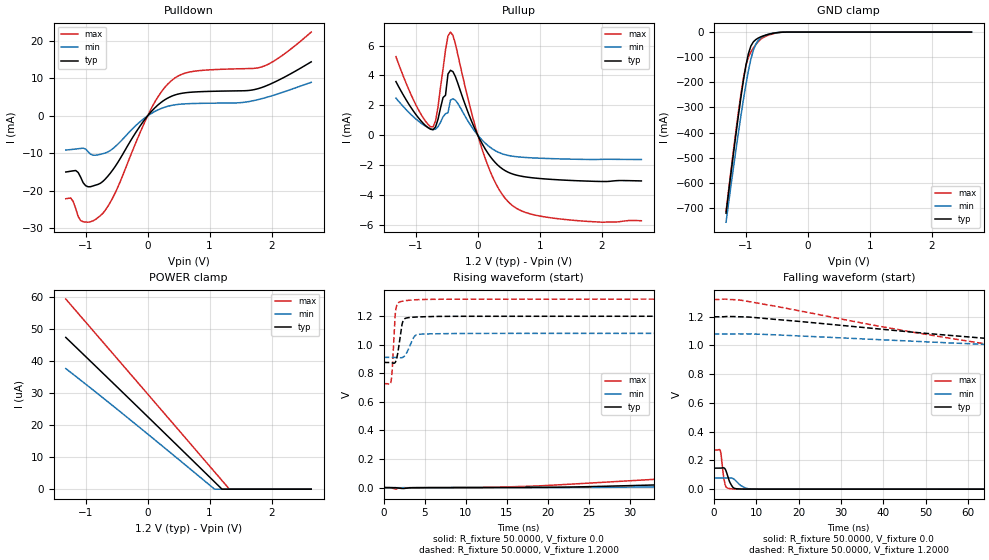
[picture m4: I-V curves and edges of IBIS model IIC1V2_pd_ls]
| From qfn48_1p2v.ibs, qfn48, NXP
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[Model] IIC1V2_pd_ls
|   Model IIC1V2_pd_ls
| This model was characterised for following simulation conditions:
| External (pad) voltage:
|   - Typ: 1.2V,   - Min: 1.08V,   - Max: 1.32V
| Library cells for typ/min/max conditions are connected as defined below:
|  IO - External Pad
|  A - Core Input
|  EN - Output Buffer Enable
|  BOOST - vdde
|  EGP - vdd
|  EHS - gnd
|  ENZI - vdd
|  EPD - vdd
|  EPUN - vdd
|  ZI - NC
|  ZIF - NC
|  gnd - gnd
|  gnde - gnde
|  vdd - vdd
|  vdde - vdde
| All other pins connected to ground
Model_type I/O
Polarity   Non-Inverting
Enable   Active-Low
Vinl =   0.5400V
Vinh =   1.2600V
Vmeas =  0.9000V
Cref =   0.0F
Rref =   1.0000k
Vref =   0.0V
C_comp   3.6164pF   3.4768pF   3.7417pF
|C_comp_pullup   0.9402pF   0.8991pF   0.9548pF
|C_comp_pulldown   2.3240pF   2.4771pF   2.1787pF
[Model Spec]
| variable   typ   min   max
Vinh   0.3600V   0.3240V   0.3960V
Vinl   0.8400V   0.7560V   0.9240V
Vmeas   0.6000V   0.5400V   0.6600V
[Temperature Range]   25.0000   0.1250k   -40.0000
[Voltage Range]   1.2000V   1.0800V   1.3200V
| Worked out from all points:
|   slope of the pulldown table from 0 to 0.18 V, typ, clamps not added: 58.3 ohm
|   slope of the pullup table from 0 to 0.18 V, typ, clamps not added: 138 ohm
|   GND clamp passes 1 mA (typ) near -0.45 V on its own axis
|   rising waveform, R_fixture 50.0000, V_fixture 0.0: 20-80 % time 73.4ns typ, 82.7ns min, 61.7ns max; typ from 0 V to 0.146 V
|   rising waveform, R_fixture 50.0000, V_fixture 1.2000: 20-80 % time 495ps typ, 789ps min, 328ps max; typ from 0.876 V to 1.2 V
|   falling waveform, R_fixture 50.0000, V_fixture 0.0: 20-80 % time 1.12ns typ, 1.9ns min, 698ps max; typ from 0.146 V to 0 V
|   falling waveform, R_fixture 50.0000, V_fixture 1.2000: 20-80 % time 83.2ns typ, 99ns min, 62.6ns max; typ from 1.2 V to 0.876 V
[Pulldown]
|Voltage   I(typ)   I(min)   I(max)
-1.32V    -14.96mA   -9.099mA   -22.09mA
-1.24V    -14.75mA   -8.982mA   -21.89mA
-1.16V    -14.56mA   -8.83mA    -24.7mA
-1.04V    -17.82mA   -8.609mA   -28.21mA
-920mV    -18.88mA   -10.21mA   -28.21mA
-720mV    -17.44mA   -10.07mA   -25.94mA
-520mV    -13.41mA   -8.157mA   -20.44mA
80mV      1.521mA    840uA      2.628mA
440mV     5.569mA    2.951mA    10.1mA
760mV     6.377mA    3.307mA    11.92mA
1.84V     7.555mA    4.581mA    13.06mA
2.64V     14.41mA    8.944mA    22.34mA
[Pullup]
|Voltage   I(typ)   I(min)   I(max)
-1.32V    3.586mA    2.482mA    5.256mA
-960mV    1.175mA    947.4uA    1.725mA
-720mV    361.5uA    375.5uA    554.5uA
-640mV    1.072mA    568.3uA    1.915mA
-520mV    2.67mA     1.432mA    5.707mA
-480mV    4.094mA    1.5mA      6.648mA
-440mV    4.341mA    2.344mA    6.901mA
120mV     -924.8uA   -536.9uA   -1.554mA
360mV     -2.143mA   -1.197mA   -3.751mA
600mV     -2.653mA   -1.434mA   -4.838mA
1.4V      -3.016mA   -1.6mA     -5.648mA
2.64V     -3.069mA   -1.636mA   -5.736mA
[GND_clamp]
|Voltage   I(typ)   I(min)   I(max)
-1.32V    -720.7mA   -756.5mA   -713.8mA
-1.12V    -330.9mA   -399.5mA   -316.8mA
-1.04V    -192.4mA   -269.2mA   -184.4mA
-1V       -133.6mA   -209.3mA   -133.5mA
-960mV    -86.74mA   -154.7mA   -99.46mA
-920mV    -55.69mA   -108.2mA   -79.02mA
-880mV    -39.02mA   -72.35mA   -63.71mA
-840mV    -29.9mA    -48mA      -50.26mA
-760mV    -18.93mA   -23.39mA   -28.32mA
-640mV    -9.22mA    -8.628mA   -12.73mA
-400mV    -335.3uA   -402.3uA   -442.6uA
2.64V     0A         0A         0A
[POWER_clamp]
|Voltage   I(typ)   I(min)   I(max)
-1.32V    47.4uA     37.67uA    59.39uA
-280mV    27.94uA    21.65uA    36.04uA
1.08V     2.274uA    0A         5.413uA
1.2V      0A         0A         2.707uA
1.32V     0A         0A         0A
2.64V     0A         0A         0A
[Ramp]
| variable   typ   min   max
dV/dt_r  87.6550m/73.3194n   46.3571m/82.7056n   0.1635/61.6982n
dV/dt_f  0.1940/83.2107n   0.1007/98.8978n   0.3551/62.5921n
R_load = 50.0000
[Rising Waveform]
R_fixture= 50.0000
V_fixture= 0.0
V_fixture_min= 0.0
V_fixture_max= 0.0
|time   V(typ)   V(min)   V(max)
0s        642.2pV    57.99nV    36.63pV
1.471ns   -816.2uV   129.4uV    -10.91mV
2.396ns   -6.561mV   -415.4uV   -655.4uV
17.81ns   1.081mV    277.8uV    9.669mV
56.15ns   53.04mV    21.26mV    131.2mV
98.91ns   104.3mV    48.28mV    227.2mV
118.7ns   120.5mV    57.43mV    250.8mV
150.2ns   135.9mV    67.39mV    265.8mV
249.6ns   145.5mV    76.3mV     272.1mV
1us       146.1mV    77.26mV    272.4mV
[Rising Waveform]
R_fixture= 50.0000
V_fixture= 1.2000
V_fixture_min= 1.0800
V_fixture_max= 1.3200
|time   V(typ)   V(min)   V(max)
0s        875.8mV    911.4mV    727.2mV
903.5ps   874mV      911.7mV    743.1mV
1.063ns   871.8mV    911.6mV    844.1mV
1.397ns   875mV      910.5mV    1.204V
1.674ns   926.7mV    909.2mV    1.286V
2.169ns   1.122V     908.3mV    1.303V
2.473ns   1.177V     916.8mV    1.306V
3.875ns   1.193V     1.065V     1.314V
6.178ns   1.197V     1.076V     1.318V
1us       1.199V     1.079V     1.319V
[Falling Waveform]
R_fixture= 50.0000
V_fixture= 0.0
V_fixture_min= 0.0
V_fixture_max= 0.0
|time   V(typ)   V(min)   V(max)
0s        146.1mV    77.29mV    272.5mV
1.542ns   146.2mV    77.3mV     268.2mV
1.729ns   146.9mV    77.28mV    238.3mV
2.311ns   148.6mV    77.22mV    89.12mV
2.906ns   126mV      77.79mV    14.79mV
4.275ns   22.45mV    76.9mV     1.973mV
5.669ns   2.09mV     43.69mV    695.3uV
7.959ns   434.8uV    3.936mV    433.2uV
12.35ns   259uV      261.6uV    245.5uV
1us       25.86nV    100.8nV    14.91nV
[Falling Waveform]
R_fixture= 50.0000
V_fixture= 1.2000
V_fixture_min= 1.0800
V_fixture_max= 1.3200
|time   V(typ)   V(min)   V(max)
0s        1.199V     1.079V     1.319V
6.611ns   1.199V     1.08V      1.314V
45.12ns   1.097V     1.032V     1.101V
69.5ns    1.037V     1.001V     985.1mV
95.31ns   983mV      974.5mV    816.9mV
113.3ns   944.4mV    959.5mV    764.9mV
136.5ns   904.2mV    943.5mV    740.5mV
171.2ns   883.1mV    926.7mV    730.7mV
248.4ns   876.8mV    914mV      727.9mV
1us       875.9mV    911.5mV    727.2mV
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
